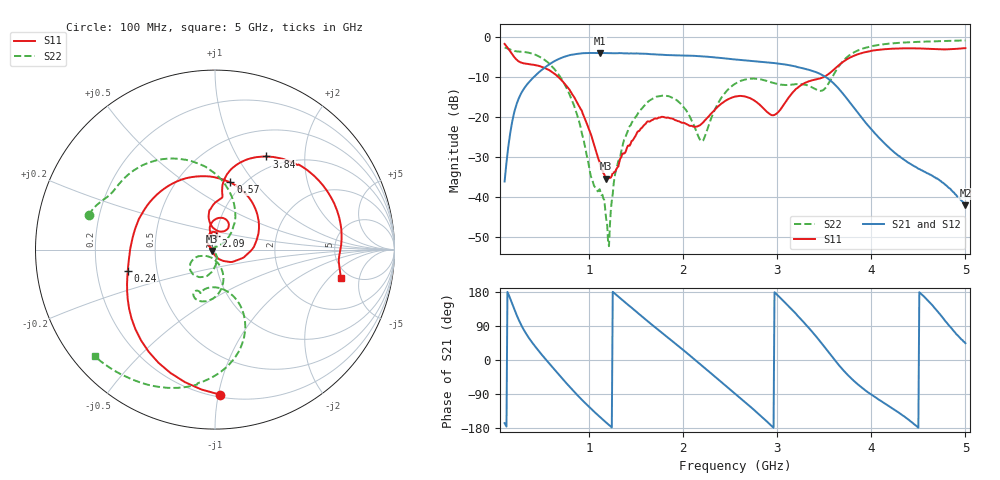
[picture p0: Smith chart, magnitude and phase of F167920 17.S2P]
!  2-Port S-parameters saved by WinCal
! VAR MeasName=S-Parameters (CALIBRATED_DATA) read from VNA (N5242A)
! VAR MeasDate=2016-11-22 9:54:26
! VAR NAME=F167920 17
! VAR FILENAME=F167920 17.S2P
! VAR DATE=2016-11-22 9:54:26
! VAR PHYS_PORTS=1,2
# Hz S DB R 50
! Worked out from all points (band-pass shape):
!   491 points, 100 MHz to 5 GHz, reference 50 ohm
!   highest |S21| = -4.09 dB at 1.11 GHz (marker M1); lowest = -42.1 dB at 5 GHz (marker M2)
!   |S21| within 3 dB of the highest: 565.5 MHz to 3.113 GHz (2.548 GHz wide, 139 % of centre)
!   lowest |S11| = -35.5 dB at 1.18 GHz (marker M3), VSWR 1.03, Z = 48.5 - j0.77 ohm
!   |S11| at or under -10 dB: 666.8 MHz to 3.502 GHz (2.835 GHz wide, 136 % of centre)
!   |S22| runs from -52.4 to -1.0 dB; largest |S21 - S12| = 0.0011
!   S11 on the Smith chart (normalised r, x): 100 MHz: 0.22, -1.01; 240 MHz: 0.34, -0.11; 570 MHz: 0.87, +0.77; 2.09 GHz: 1.00, +0.15; 3.84 GHz: 0.83, +1.33; 5 GHz: 4.22, -2.75
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1e8  -1.84 -88.0  -36.20 -166.7  -36.16 -167.0  -2.74 164.7
1.7e8  -4.05 -135.0  -22.63 155.8  -22.63 155.7  -3.34 155.9
2.4e8  -6.02 -166.5  -16.05 111.7  -16.05 111.7  -3.71 149.5
4.3e8  -7.13 126.1  -9.67 34.2  -9.66 34.2  -4.56 122.3
5.7e8  -8.31 77.1  -7.01 -7.7  -7.02 -7.7  -6.64 96.6
7.2e8  -11.26 26.4  -5.18 -50.9  -5.18 -50.9  -11.15 67.5
9.2e8  -18.47 -35.0  -4.16 -104.3  -4.16 -104.3  -24.05 37.6
1.11e9  -31.27 -101.5  -4.09 -149.5  -4.09 -149.5  -38.13 126.1
1.18e9  -35.51 -151.8  -4.13 -165.0  -4.13 -165.0  -45.59 146.7
1.21e9  -35.36 -174.6  -4.14 -171.5  -4.14 -171.5  -52.36 -123.9
1.28e9  -33.56 160.9  -4.16 173.7  -4.16 173.7  -33.80 -80.3
1.41e9  -27.27 145.2  -4.18 146.1  -4.18 146.1  -23.58 -80.2
1.74e9  -20.21 100.9  -4.50 78.4  -4.51 78.3  -14.90 -124.5
2.09e9  -22.31 85.5  -4.77 7.7  -4.77 7.7  -21.01 -156.0
2.21e9  -21.47 101.7  -4.96 -17.3  -4.96 -17.3  -25.98 -105.3
2.55e9  -14.98 82.8  -5.70 -88.5  -5.72 -88.5  -11.81 -88.1
2.96e9  -19.64 78.7  -6.59 -178.9  -6.60 -178.8  -11.59 -116.1
3.37e9  -10.92 84.0  -8.54 74.7  -8.56 74.7  -12.68 -105.6
3.55e9  -9.26 83.3  -10.69 19.1  -10.71 19.1  -11.50 -70.0
3.84e9  -4.54 61.1  -18.55 -60.8  -18.58 -60.7  -3.64 -84.4
4.19e9  -3.07 29.2  -27.79 -122.4  -27.83 -121.9  -1.76 -109.6
5e9  -2.88 -12.7  -42.14 44.3  -41.91 44.5  -0.96 -138.4
